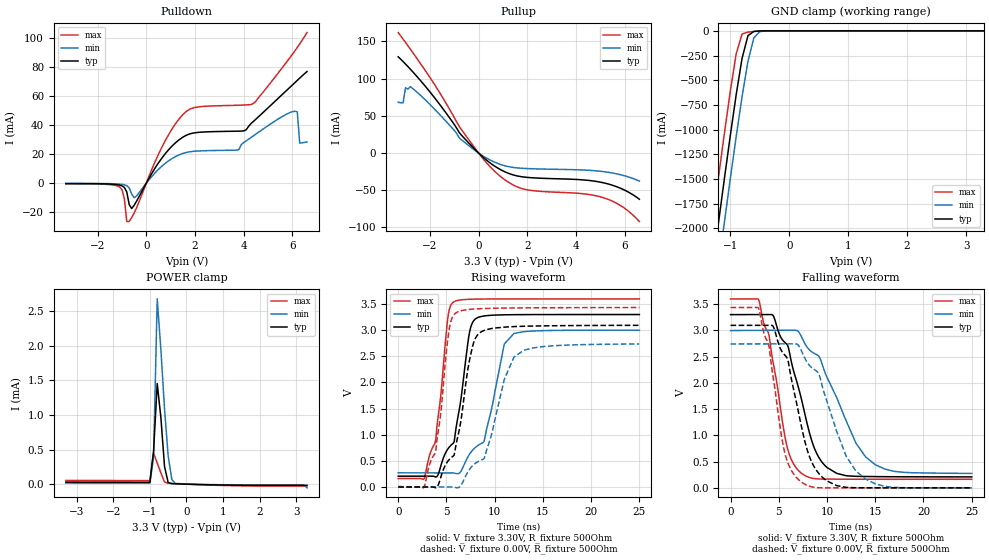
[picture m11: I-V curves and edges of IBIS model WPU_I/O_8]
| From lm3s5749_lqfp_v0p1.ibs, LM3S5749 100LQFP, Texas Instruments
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[Model]   WPU_I/O_8
Model_type   I/O
Vinl = 1.26
Vinh = 2.04
Vmeas = 1.65
| variable   typ   min   max
C_comp   9.739pF   9.739pF   9.803pF
[Model Spec]
Vinh+   1.91   1.78   2.04
Vinh-   1.90   1.76   2.03
Vinl+   1.40   1.27   1.54
Vinl-   1.39   1.26   1.53
| variable   typ   min   max
[Temperature Range]  25   85   -40
[Voltage Range]   3.3V   3.0V   3.6V
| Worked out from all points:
|   slope of the pulldown table from 0 to 0.495 V, typ, clamps not added: 35.8 ohm
|   slope of the pullup table from 0 to 0.495 V, typ, clamps not added: 35.8 ohm
|   GND clamp passes 1 mA (typ) near -0.48 V on its own axis
|   POWER clamp passes 1 mA (typ) near -0.71 V on its own axis
|   falling waveform, V_fixture 3.30V, R_fixture 500Ohm: 20-80 % time 2.57ns typ, 3.82ns min, 1.8ns max; typ from 3.3 V to 0.208 V
|   rising waveform, V_fixture 3.30V, R_fixture 500Ohm: 20-80 % time 1.54ns typ, 2.24ns min, 1.14ns max; typ from 0.208 V to 3.3 V
|   falling waveform, V_fixture 0.00V, R_fixture 500Ohm: 20-80 % time 2.29ns typ, 3.1ns min, 1.68ns max; typ from 3.09 V to 0 V
|   rising waveform, V_fixture 0.00V, R_fixture 500Ohm: 20-80 % time 1.64ns typ, 2.39ns min, 1.21ns max; typ from 0 V to 3.09 V
[Pulldown]
|  Voltage   I(typ)   I(min)   I(max)
-3.3V     -256.4uA   -145.5uA   -364.3uA
-1.1V     -1.272mA   -586.9uA   -2.565mA
-700mV    -14.71mA   -3.213mA   -26.31mA
-500mV    -15.24mA   -9.997mA   -20.64mA
600mV     16.38mA    11.14mA    23.43mA
1.5V      31.7mA     20.53mA    47.23mA
3.8V      35.88mA    23.14mA    53.74mA
4.4V      42.6mA     32.69mA    54.97mA
6.1V      69.26mA    49.6mA     91.12mA
6.2V      70.84mA    49.17mA    93.51mA
6.3V      72.42mA    27.66mA    95.98mA
6.6V      76.89mA    28.41mA    103.8mA
[Pullup]
|  Voltage   I(typ)   I(min)   I(max)
-3.3V     129.3mA    68.2mA     161.9mA
-3.1V     122.9mA    67.41mA    153.1mA
-3V       119.6mA    87.83mA    148.7mA
-2.8V     112.7mA    89.21mA    139.6mA
-1.8V     73.98mA    58.72mA    91.66mA
-700mV    23.82mA    17.72mA    31.27mA
300mV     -8.84mA    -6.3mA     -12.15mA
1V        -23.98mA   -16.37mA   -34.08mA
2V        -32.71mA   -20.86mA   -49.43mA
5.1V      -39.81mA   -24.88mA   -59.77mA
5.9V      -48.4mA    -29.75mA   -72.06mA
6.6V      -62.06mA   -37.61mA   -92.08mA
[GND Clamp]
|  Voltage   I(typ)   I(min)   I(max)
-3.3V     -11.73A    -12.14A    -11.32A
-1.4V     -2.85A     -3.29A     -2.391A
-1.3V     -2.393A    -2.835A    -1.933A
-1.2V     -1.942A    -2.383A    -1.481A
-1.1V     -1.496A    -1.937A    -1.038A
-1V       -1.061A    -1.498A    -612.1mA
-900mV    -646.5mA   -1.071A    -233.9mA
-800mV    -278.2mA   -665.9mA   -32.19mA
-700mV    -49.13mA   -307.7mA   -12.51mA
-600mV    -5.771mA   -70.87mA   -6.526mA
-500mV    -1.221mA   -8.174mA   -2.28mA
3.3V      2.312nA    7.026uA    -6.841uA
[POWER Clamp]
|  Voltage   I(typ)   I(min)   I(max)
-3.3V     29.71uA    15.87uA    54.94uA
-1V       27.67uA    14.78uA    51.22uA
-900mV    477.6uA    387.3uA    449.4uA
-800mV    1.453mA    2.675mA    305uA
-700mV    962.1uA    1.944mA    163.7uA
-600mV    254.6uA    1.086mA    31.4uA
-500mV    22.38uA    405.6uA    14.49uA
-400mV    7.783uA    67.02uA    10.49uA
-300mV    5.498uA    7.026uA    7.722uA
3.1V      -16.64uA   -9.952uA   -27.43uA
3.2V      -16.65uA   -12.25uA   -27.44uA
3.3V      -16.65uA   -53.27uA   -27.45uA
[Ramp]
| variable   typ   min   max
dV/dt_f   1.85/2.57n   1.63/3.82n   2.06/1.80n
dV/dt_r   1.86/1.64n   1.63/2.39n   2.06/1.21n
R_load = 500Ohm
[Falling Waveform]
V_fixture = 3.30V
V_fixture_min = 3.00V
V_fixture_max = 3.60V
R_fixture = 500Ohm
|   Time   V(typ)   V(min)   V(max)
0s        3.298V     2.994V     3.597V
2.9ns     3.298V     2.998V     3.588V
4ns       3.298V     2.998V     2.898V
5.9ns     2.717V     2.999V     754.8mV
7.4ns     1.65V      2.859V     271.3mV
8.6ns     799.3mV    2.568V     178.4mV
9.8ns     422.5mV    2.192V     166.9mV
13ns      219mV      852mV      163.9mV
15ns      214mV      441.3mV    163.3mV
25ns      208.2mV    274.5mV    162.3mV
[Rising Waveform]
V_fixture = 3.30V
V_fixture_min = 3.00V
V_fixture_max = 3.60V
R_fixture = 500Ohm
|   Time   V(typ)   V(min)   V(max)
0s        207.6mV    271.4mV    162.2mV
2.7ns     207.4mV    270.4mV    165.3mV
3.9ns     191.8mV    270.1mV    914mV
5.1ns     714.8mV    269.9mV    3.171V
5.7ns     836.9mV    269.3mV    3.533V
7.4ns     2.965V     630.1mV    3.591V
8.1ns     3.227V     771.5mV    3.594V
11ns      3.294V     2.736V     3.597V
12ns      3.296V     2.937V     3.597V
25ns      3.299V     2.999V     3.598V
[Falling Waveform]
V_fixture = 0.00V
V_fixture_min = 0.00V
V_fixture_max = 0.00V
R_fixture = 500Ohm
|   Time   V(typ)   V(min)   V(max)
0s        3.093V     2.739V     3.433V
2.9ns     3.093V     2.74V      3.423V
4ns       3.094V     2.741V     2.68V
5.6ns     2.532V     2.741V     685.6mV
7.3ns     1.21V      2.629V     116.7mV
8.2ns     586.3mV    2.327V     30.35mV
9.4ns     222.8mV    2.013V     1.741mV
12ns      7.855mV    597.6mV    107.7uV
14ns      1.389mV    166.7mV    70.3uV
25ns      37.48uV    42.83uV    16.46uV
[Rising Waveform]
V_fixture = 0.00V
V_fixture_min = 0.00V
V_fixture_max = 0.00V
R_fixture = 500Ohm
|   Time   V(typ)   V(min)   V(max)
0s        365.8uV    12.24mV    108.2uV
2.7ns     122.3uV    1.727mV    4.268mV
3.9ns     -14.91mV   677.3uV    699.6mV
5.2ns     506.2mV    277.7uV    2.901V
5.9ns     711.2mV    -6.26mV    3.319V
7.5ns     2.521V     363.7mV    3.399V
8.5ns     2.956V     507.8mV    3.411V
9ns       3.001V     598.7mV    3.414V
12ns      3.068V     2.484V     3.425V
25ns      3.092V     2.736V     3.432V
